|TEXAS INSTRUMENTS INCORPORATED
|Standard Linear and Logic
|IBIS Model of SN74ACT374
|OCTAL D-TYPE EDGE-TRIGGERED FLIP-FLOPS WITH 3-STATE OUTPUTS
|SOIC 20-pin (DW), SOP 20-pin (NS)SSOP 20-pin (DB) TSSOP 20-pin (PW),
|PDIP 20-pin (N) packages.
[IBIS Ver]   3.2
[Comment Char]  |_char
[File Name]   sn74act374.ibs
[File Rev]   1.1
[Date]   10/28/04
[Source]   File originated at Texas Instruments, Inc.
[Notes]   The following is a sample IBIS file for the ACT374.
   - FILE REV HISTORY
   - 1.1 Release IBIS file on 11/02/04
|   - All test data contained in this file are derived from
|   actual measurement.
|   - The measurement used NS package.
|   - We have data across voltage and temperature, but not across
|   process.
|*   Property of Texas Instruments Incorporated.  Unauthorized   *
|*   reproduction and/or distribution is strictly prohibited.   *
|*   This product is protected under copyright law.   *
|*   Created 1998, (C) Copyright 1998, Texas Instruments Inc.,   *
|*   All Rights Reserved   *
|*   UNLESS THERE IS A SIGNED, WRITTEN AGREEMENT TO THE   *
|*   CONTRARY, TEXAS INSTRUMENTS ("TI") IS PROVIDING THE SPICE   *
|*   MODELS "AS IS" AND WITHOUT ANY WARRANTY, EXPRESSED OR   *
|*   IMPLIED.  TI assumes no liability for:   *
|*   1) the accuracy of the IBIS models provided to your   *
|*   company;   *
|*   2) the proper functioning of these IBIS models in your   *
|*   design or for any resulting applications; or   *
|*   3) infringement of patents, copyrights or intellectual   *
|*   property rights resulting from your use of these   *
|*   IBIS models.   *
|*   TI provides IBIS Models as a service to our customers.   *
|*   You and your company shall not distribute, sell or give   *
|*   these models to anyone else without prior written   *
|*   permission from TI.   *
|*   TI reserves the right to make changes to our products or   *
|*   to discontinue any semiconductor product or service   *
|*   without notice, and advises our customers to obtain the   *
|*   latest version of relevant information to verify, before   *
|*   placing orders, that the information being relied on is   *
|*   current.   *
|*   Please be aware that your receipt and use of the IBIS   *
|*   information provided shall serve as acceptance of these   *
|*   terms and conditions.  If you do not accept these terms,   *
|*   you should return or destroy the IBIS models and any   *
|*   other accompanying information immediately.   *
|   Component ACT374_DW
[Component]   ACT374_DW
[Manufacturer]  Texas Instruments, Inc.
[Package]
|   typ   min   max
R_pkg   0.038   0.033   0.045
L_pkg   5.012nH   4.110nH   6.349nH
C_pkg   0.717pF   0.530pF   0.868pF
[Pin]  signal_name  model_name   R_pin   L_pin   C_pin
1   OE_BAR   ACT374_NC   0.042   6.336nH   0.865pF
2   1Q   ACT374_OUT   0.043   5.542nH   0.867pF
3   1D   ACT374_IN   0.034   4.714nH   0.732pF
4   2D   ACT374_IN   0.034   4.377nH   0.591pF
5   2Q   ACT374_OUT   0.036   4.130nH   0.533pF
6   3Q   ACT374_OUT   0.035   4.111nH   0.530pF
7   3D   ACT374_IN   0.034   4.284nH   0.583pF
8   4D   ACT374_IN   0.034   4.634nH   0.726pF
9   4Q   ACT374_OUT   0.040   5.518nH   0.865pF
10   GND   GND   0.043   6.349nH   0.866pF
11   CLK   ACT374_NC   0.041   6.281nH   0.861pF
12   5Q   ACT374_OUT   0.045   5.561nH   0.868pF
13   5D   ACT374_IN   0.033   4.778nH   0.742pF
14   6D   ACT374_IN   0.035   4.414nH   0.596pF
15   6Q   ACT374_OUT   0.035   4.110nH   0.533pF
16   7Q   ACT374_OUT   0.036   4.130nH   0.533pF
17   7D   ACT374_IN   0.034   4.377nH   0.591pF
18   8D   ACT374_IN   0.034   4.714nH   0.731pF
19   8Q   ACT374_NC   0.043   5.569nH   0.868pF
20   VCC   POWER   0.042   6.308nH   0.864pF
|   Component ACT374_NS
[Component]   ACT374_NS
[Manufacturer]  Texas Instruments, Inc.
[Package]
|   typ   min   max
R_pkg   0.044   0.029   0.058
L_pkg   3.666nH   2.317nH   5.115nH
C_pkg   0.548pF   0.316pF   0.725pF
[Pin]  signal_name  model_name   R_pin   L_pin   C_pin
1   OE_BAR   ACT374_NC   0.058   5.115nH   0.725pF
2   1Q   ACT374_OUT   0.053   4.591nH   0.724pF
3   1D   ACT374_IN   0.049   3.754nH   0.572pF
4   2D   ACT374_IN   0.029   2.549nH   0.388pF
5   2Q   ACT374_OUT   0.031   2.317nH   0.316pF
6   3Q   ACT374_OUT   0.031   2.317nH   0.316pF
7   3D   ACT374_IN   0.029   2.556nH   0.399pF
8   4D   ACT374_IN   0.049   3.754nH   0.579pF
9   4Q   ACT374_OUT   0.053   4.591nH   0.724pF
10   GND   GND   0.058   5.115nH   0.725pF
11   CLK   ACT374_NC   0.058   5.115nH   0.725pF
12   5Q   ACT374_OUT   0.053   4.591nH   0.724pF
13   5D   ACT374_IN   0.049   3.754nH   0.579pF
14   6D   ACT374_IN   0.029   2.557nH   0.399pF
15   6Q   ACT374_OUT   0.031   2.317nH   0.316pF
16   7Q   ACT374_OUT   0.031   2.317nH   0.316pF
17   7D   ACT374_IN   0.029   2.557nH   0.399pF
18   8D   ACT374_IN   0.049   3.754nH   0.579pF
19   8Q   ACT374_NC   0.053   4.591nH   0.724pF
20   VCC   POWER   0.058   5.115nH   0.725pF
|   Component ACT374_DB
[Component]   ACT374_DB
[Manufacturer]  Texas Instruments, Inc.
[Package]
|   typ   min   max
R_pkg   0.040   0.035   0.051
L_pkg   3.495nH   3.035nH   4.314nH
C_pkg   0.420pF   0.346pF   0.502pF
[Pin]  signal_name  model_name   R_pin   L_pin   C_pin
1   OE_BAR   ACT374_NC   0.049   4.310nH   0.502pF
2   1Q   ACT374_OUT   0.048   3.903nH   0.487pF
3   1D   ACT374_IN   0.035   3.189nH   0.396pF
4   2D   ACT374_IN   0.035   3.036nH   0.347pF
5   2Q   ACT374_OUT   0.035   3.035nH   0.367pF
6   3Q   ACT374_OUT   0.035   3.035nH   0.367pF
7   3D   ACT374_IN   0.035   3.036nH   0.347pF
8   4D   ACT374_IN   0.035   3.189nH   0.397pF
9   4Q   ACT374_OUT   0.047   3.899nH   0.488pF
10   GND   GND   0.051   4.314nH   0.500pF
11   CLK   ACT374_NC   0.051   4.314nH   0.500pF
12   5Q   ACT374_OUT   0.047   3.899nH   0.488pF
13   5D   ACT374_IN   0.035   3.189nH   0.397pF
14   6D   ACT374_IN   0.035   3.036nH   0.346pF
15   6Q   ACT374_OUT   0.035   3.035nH   0.367pF
16   7Q   ACT374_OUT   0.035   3.035nH   0.367pF
17   7D   ACT374_IN   0.035   3.036nH   0.346pF
18   8D   ACT374_IN   0.035   3.189nH   0.397pF
19   8Q   ACT374_NC   0.047   3.899nH   0.488pF
20   VCC   POWER   0.051   4.314nH   0.502pF
|   Component ACT374_PW
[Component]   ACT374_PW
[Manufacturer]  Texas Instruments, Inc.
[Package]
|   typ   min   max
R_pkg   0.035   0.024   0.047
L_pkg   2.399nH   1.710nH   3.250nH
C_pkg   0.284pF   0.166pF   0.418pF
[Pin]  signal_name  model_name   R_pin   L_pin   C_pin
1   OE_BAR   ACT374_NC   0.041   3.102nH   0.410pF
2   1Q   ACT374_OUT   0.040   2.777nH   0.363pF
3   1D   ACT374_IN   0.029   2.194nH   0.260pF
4   2D   ACT374_IN   0.025   1.710nH   0.166pF
5   2Q   ACT374_OUT   0.025   1.740nH   0.191pF
6   3Q   ACT374_OUT   0.024   1.763nH   0.193pF
7   3D   ACT374_IN   0.024   1.817nH   0.174pF
8   4D   ACT374_IN   0.028   2.256nH   0.265pF
9   4Q   ACT374_OUT   0.045   2.887nH   0.368pF
10   GND   GND   0.047   3.250nH   0.417pF
11   CLK   ACT374_NC   0.046   3.244nH   0.418pF
12   5Q   ACT374_OUT   0.046   2.961nH   0.375pF
13   5D   ACT374_IN   0.033   2.334nH   0.268pF
14   6D   ACT374_IN   0.029   1.915nH   0.179pF
15   6Q   ACT374_OUT   0.031   1.934nH   0.203pF
16   7Q   ACT374_OUT   0.032   1.917nH   0.201pF
17   7D   ACT374_IN   0.030   1.833nH   0.173pF
18   8D   ACT374_IN   0.036   2.324nH   0.268pF
19   8Q   ACT374_NC   0.042   2.869nH   0.372pF
20   VCC   POWER   0.042   3.160nH   0.414pF
|   Component ACT374_N
[Component]   ACT374_N
[Manufacturer]   Texas Instruments, Inc.
[Package]
|   typ   min   max
R_pkg   4.300e-02   3.800e-02   5.000e-02
L_pkg   7.384e-09   4.680e-09   1.032e-08
C_pkg   5.100e-13   2.310e-13   8.210e-13
[Pin]   signal_name   model_name   R_pin   L_pin   C_pin
1   OE_BAR   ACT374_NC   4.200e-02   9.427e-09   8.100e-13
2   1Q   ACT374_OUT   4.600e-02   8.544e-09   4.560e-13
3   1D   ACT374_IN   4.800e-02   7.163e-09   4.350e-13
4   2D   ACT374_IN   4.000e-02   4.825e-09   2.610e-13
5   2Q   ACT374_OUT   4.000e-02   5.284e-09   6.480e-13
6   3Q   ACT374_OUT   4.000e-02   4.686e-09   2.320e-13
7   3D   ACT374_IN   4.000e-02   6.359e-09   4.890e-13
8   4D   ACT374_IN   3.800e-02   7.982e-09   4.750e-13
9   4Q   ACT374_OUT   4.300e-02   9.403e-09   4.750e-13
10   GND   GND   5.000e-02   1.032e-08   8.050e-13
11   CLK   ACT374_NC   5.000e-02   1.028e-08   8.100e-13
12   5Q   ACT374_OUT   4.300e-02   9.383e-09   4.770e-13
13   5D   ACT374_IN   3.800e-02   7.978e-09   4.760e-13
14   6D   ACT374_IN   4.000e-02   6.302e-09   4.920e-13
15   6Q   ACT374_OUT   4.000e-02   4.680e-09   2.310e-13
16   7Q   ACT374_OUT   4.000e-02   5.284e-09   6.480e-13
17   7D   ACT374_IN   4.000e-02   4.822e-09   2.610e-13
18   8D   ACT374_IN   4.700e-02   7.118e-09   4.390e-13
19   8Q   ACT374_OUT   4.600e-02   8.492e-09   4.610e-13
20   VCC   POWER   4.300e-02   9.348e-09   8.210e-13
| Models and submodels in the file (3): ACT374_IN (Input), ACT374_NC (Input), ACT374_OUT (3-state)
